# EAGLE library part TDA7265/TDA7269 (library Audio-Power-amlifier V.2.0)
The TDA7265 is class AB dual Audio power amplifier assembled in the Multiwatt package, specially designed for high quality sound application as Hi-Fi music centers and stereo TV sets
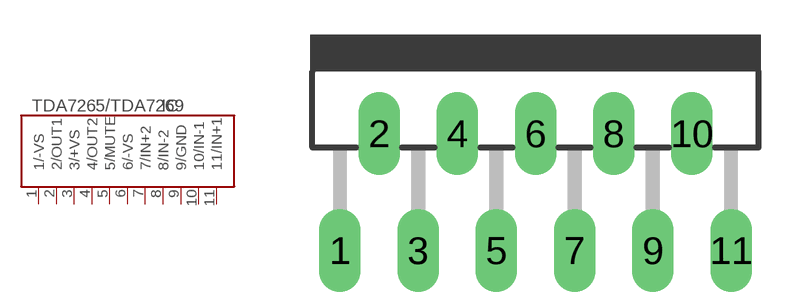
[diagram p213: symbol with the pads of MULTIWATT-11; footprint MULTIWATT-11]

Designator prefix IC

## TDA7265/TDA7269  [MULTIWATT-11]
1  1/-VS  pwr
2  2/OUT1  out
3  3/+VS  pwr
4  4/OUT2  out
5  5/MUTE  in
6  6/-VS  pwr
7  7/IN+2  in
8  8/IN-2  in
9  9/GND  pwr
10  10/IN-1  in
11  11/IN+1  in

## Footprint MULTIWATT-11 (pad centres in mm)
Muliwatt 11 lead
drill 1.2 long: 1 -8.5,-6.35; 2 -6.8,-1.27; 3 -5.1,-6.35; 4 -3.4,-1.27; 5 -1.7,-6.35; 6 0,-1.27; 7 1.7,-6.35; 8 3.4,-1.27; 9 5.1,-6.35; 10 6.8,-1.27; 11 8.5,-6.35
